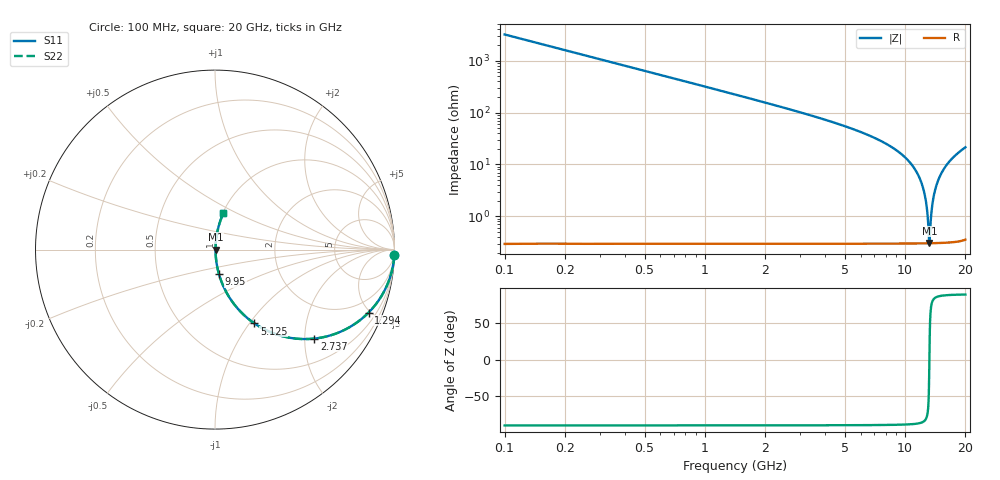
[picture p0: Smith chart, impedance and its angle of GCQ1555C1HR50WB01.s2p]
!Murata Part Number: GCQ1555C1HR50WB01
!These Parameters are Measured in Series Mode Connection
!Data Generated on Mar 13, 2026
!  o--ll--o
!Port1  Port2
!  o------o
!Operation Temp=25[degC], DC Bias Voltage=0[V]
!Freq. Start=100[MHz] Stop=20[GHz] 401[Steps]
# Hz S RI R 50
!Freq.(Hz) S11(Real) S11(Imag) S21(Real) S21(Imag) S12(Real) S12(Imag) S22(Real) S22(Imag)
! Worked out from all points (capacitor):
!   401 points, 100 MHz to 20 GHz, reference 50 ohm
!   read as one part in series: C = 500 fF near 199.5 MHz
!   lowest |Z| = 309 mohm at 13.23 GHz (marker M1)
!   series resonance near 13.22 GHz, so ESL is about 290 pH
!   S11 on the Smith chart (normalised r, x): 100 MHz: 1, -64; 1.294 GHz: 1.01, -4.87; 2.737 GHz: 1.01, -2.23; 5.125 GHz: 1.01, -1.06; 9.95 GHz: 1.01, -0.28; 20 GHz: 1.01, +0.43
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1e8  0.999 -0.0314  0.000989 0.0314  0.000989 0.0314  0.999 -0.0314
2.99e8  0.9912 -0.0932  0.00878 0.0932  0.00878 0.0932  0.9912 -0.0932
5.4775e8  0.9711 -0.1674  0.0289 0.1674  0.0289 0.1674  0.9711 -0.1674
1.294e9  0.8555 -0.351  0.1445 0.351  0.1445 0.351  0.8555 -0.351
2.73675e9  0.5534 -0.4958  0.4466 0.4958  0.4466 0.4958  0.5534 -0.4958
3.43325e9  0.4283 -0.4931  0.5717 0.4931  0.5717 0.4931  0.4283 -0.4931
5.12475e9  0.2196 -0.4111  0.7804 0.4111  0.7804 0.4111  0.2196 -0.4111
6.7665e9  0.11 -0.3087  0.89 0.3087  0.89 0.3087  0.11 -0.3087
9.9505e9  0.0219 -0.1358  0.9781 0.1358  0.9781 0.1358  0.0219 -0.1358
1.005e10  0.0206 -0.1312  0.9794 0.1312  0.9794 0.1312  0.0206 -0.1312
1.139325e10  0.00816 -0.0715  0.9918 0.0715  0.9918 0.0715  0.00816 -0.0715
1.228875e10  0.00426 -0.0352  0.9957 0.0352  0.9957 0.0352  0.00426 -0.0352
1.278625e10  0.00328 -0.0161  0.9967 0.0161  0.9967 0.0161  0.00328 -0.0161
1.29355e10  0.00313 -0.0105  0.9969 0.0105  0.9969 0.0105  0.00313 -0.0105
1.31345e10  0.00304 -0.0031  0.997 0.0031  0.997 0.0031  0.00304 -0.0031
1.3234e10  0.00303 0.000548  0.997 -0.000548  0.997 -0.000548  0.00303 0.000548
1.338325e10  0.00307 0.00597  0.9969 -0.00597  0.9969 -0.00597  0.00307 0.00597
1.37315e10  0.00338 0.0184  0.9966 -0.0184  0.9966 -0.0184  0.00338 0.0184
1.43285e10  0.00458 0.039  0.9954 -0.039  0.9954 -0.039  0.00458 0.039
1.527375e10  0.00803 0.0701  0.992 -0.0701  0.992 -0.0701  0.00803 0.0701
1.67165e10  0.0164 0.1141  0.9836 -0.1141  0.9836 -0.1141  0.0164 0.1141
2e10  0.0469 0.2032  0.9531 -0.2032  0.9531 -0.2032  0.0469 0.2032
